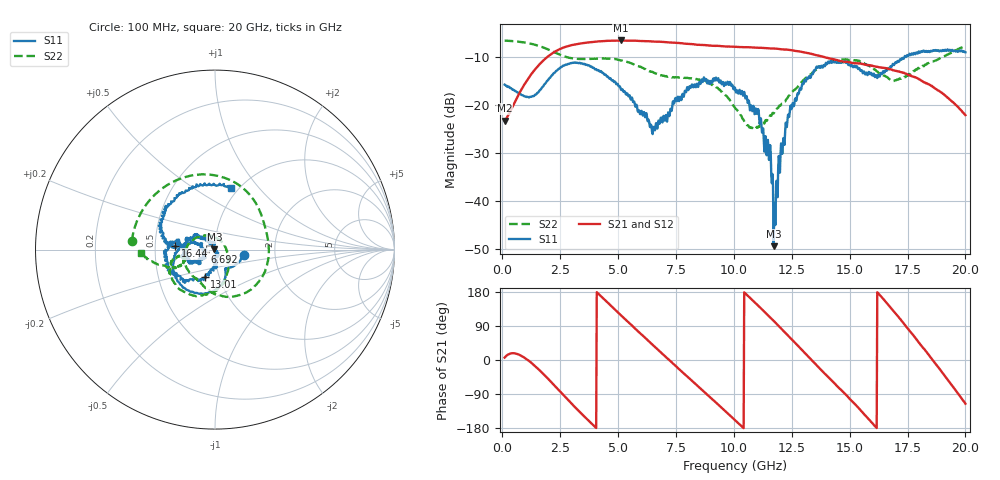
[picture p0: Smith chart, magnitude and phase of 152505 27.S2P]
!  2-Port S-parameters saved by WinCal
! VAR MeasName=S-Parameters (CALIBRATED_DATA) read from VNA (N5230C)
! VAR MeasDate=4/10/2015 9:31:01 AM
! VAR NAME=152505 27
! VAR FILENAME=152505 27.S2P
! VAR DATE=4/10/2015 9:31:01 AM
! VAR PHYS_PORTS=1,2
# Hz S DB R 50
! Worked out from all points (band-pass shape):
!   801 points, 100 MHz to 20 GHz, reference 50 ohm
!   highest |S21| = -6.60 dB at 5.125 GHz (marker M1); lowest = -23.3 dB at 100 MHz (marker M2)
!   |S21| within 3 dB of the highest: 2.062 GHz to 13.51 GHz (11.45 GHz wide, 147 % of centre)
!   lowest |S11| = -49.5 dB at 11.72 GHz (marker M3), VSWR 1.01, Z = 49.7 + j0.133 ohm
!   |S11| at or under -10 dB: start of sweep to 17.37 GHz; 17.42165 GHz to 17.44356 GHz (21.91 MHz wide, 0.126 % of centre)
!   |S22| runs from -25.1 to -6.6 dB; largest |S21 - S12| = 0.0073
!   S11 on the Smith chart (normalised r, x): 100 MHz: 1.38, -0.08; 6.692 GHz: 0.90, -0.02; 13.01 GHz: 0.85, -0.27; 16.44 GHz: 0.64, +0.03; 20 GHz: 0.92, +0.72
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1e8  -15.80 -10.4  -23.28 6.3  -23.25 6.4  -6.64 174.0
1.04525e9  -18.38 -59.1  -15.09 2.5  -15.08 2.4  -7.10 118.1
1.891e9  -15.35 -71.4  -10.25 -44.1  -10.25 -44.2  -8.29 70.5
3.43325e9  -11.37 -144.1  -7.19 -142.4  -7.19 -142.4  -10.46 8.2
4.254125e9  -12.98 -175.0  -6.76 168.7  -6.75 168.5  -10.34 -23.3
5.12475e9  -16.87 166.7  -6.60 117.9  -6.67 117.8  -10.79 -59.4
6.691875e9  -24.98 -166.5  -6.85 29.2  -6.84 29.2  -13.56 -109.1
6.741625e9  -23.30 -166.7  -6.86 26.2  -6.86 26.0  -13.72 -110.5
8.5575e9  -15.68 -167.3  -7.52 -75.2  -7.49 -75.1  -14.90 -159.2
1.005e10  -16.46 155.7  -7.92 -158.7  -7.93 -158.9  -20.65 121.3
1.106988e10  -21.12 131.8  -8.12 142.2  -8.08 142.0  -24.47 14.3
1.156738e10  -28.41 101.5  -8.26 112.3  -8.23 112.4  -22.22 -23.3
1.171662e10  -49.47 156.6  -8.28 103.4  -8.29 103.0  -21.82 -30.3
1.181612e10  -39.45 -102.2  -8.30 97.2  -8.33 96.9  -21.15 -35.1
1.23385e10  -22.10 -89.2  -8.53 64.7  -8.58 64.3  -18.41 -53.3
1.301012e10  -15.66 -110.7  -9.05 22.2  -9.04 22.2  -14.83 -71.2
1.338325e10  -13.54 -125.1  -9.45 -1.5  -9.41 -1.4  -13.33 -84.2
1.477625e10  -10.96 -178.3  -11.02 -87.8  -11.02 -88.5  -10.54 -133.7
1.644288e10  -13.00 174.8  -12.31 161.7  -12.17 161.6  -13.84 -169.8
1.669162e10  -12.56 177.2  -12.51 143.8  -12.54 142.9  -14.56 -166.9
1.828362e10  -8.82 135.7  -15.43 23.7  -15.43 23.9  -11.66 -157.6
2e10  -9.05 75.6  -22.16 -115.3  -22.22 -114.3  -7.68 -177.1
